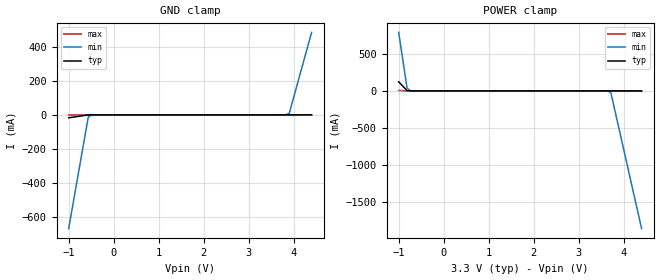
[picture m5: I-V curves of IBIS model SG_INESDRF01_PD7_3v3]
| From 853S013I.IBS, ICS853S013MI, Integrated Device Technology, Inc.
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[Model] SG_INESDRF01_PD7_3v3
Model_type   Input
Polarity   Non-Inverting
Vinl = 0.8V
Vinh = 2.0V
|   typ   min   max
C_comp   2pF   1.5pF   2.5pF
|   typ   min   max
[Voltage range]   3.3V   3.135V   3.465V
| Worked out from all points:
|   GND clamp passes 1 mA (typ) near -0.58 V on its own axis
|   POWER clamp passes 1 mA (typ) near -0.76 V on its own axis
[GND_clamp]
|Voltage   I (typ)   I (min)   I (max)
-999mV    -17.25mA   -669.4mA   -57.61uA
-564.6mV  -245.6uA   -14.47mA   -7.295uA
-502.5mV  -27.9uA    -1.943mA   -6.234uA
-378.4mV  -5.16uA    -39.86uA   -4.684uA
3.841V    50.75uA    1.283mA    47.55uA
3.904V    52.59uA    9.247mA    48.31uA
4.4V      150.7uA    485.1mA    54.46uA
[Power_clamp]
|Voltage   I (typ)   I (min)   I (max)
-999mV    122.4mA    788mA      6.109mA
-812.8mV  3.927mA    38.66mA    147.8uA
-750.8mV  399.4uA    5.222mA    56.5uA
3.593V    -3.873uA   -467.3uA   -1.587uA
3.655V    -4.754uA   -3.451mA   -2.355uA
3.717V    -6.276uA   -25.73mA   -3.124uA
4.4V      -102uA     -1.856A    -11.57uA
